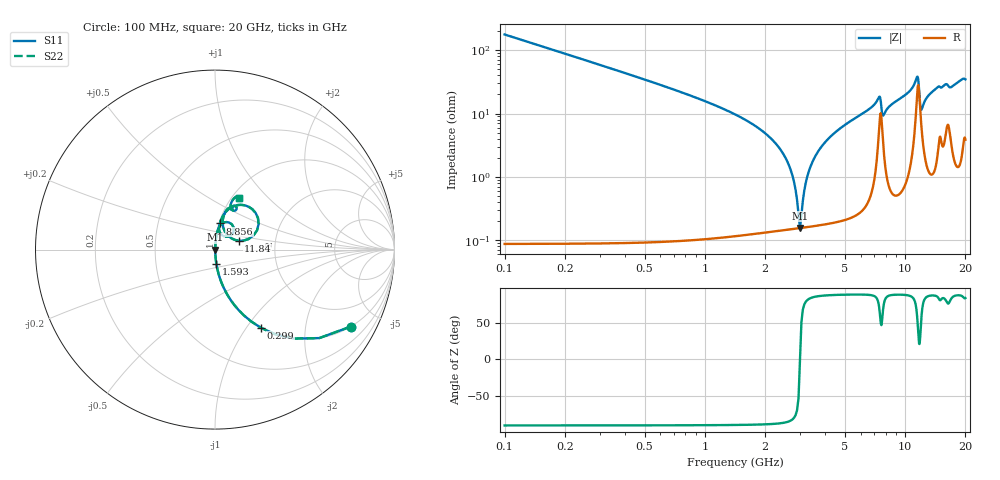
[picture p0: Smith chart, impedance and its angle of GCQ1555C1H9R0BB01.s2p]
!Murata Part Number: GCQ1555C1H9R0BB01
!These Parameters are Measured in Series Mode Connection
!Data Generated on Mar 13, 2026
!  o--ll--o
!Port1  Port2
!  o------o
!Operation Temp=25[degC], DC Bias Voltage=0[V]
!Freq. Start=100[MHz] Stop=20[GHz] 401[Steps]
# Hz S RI R 50
!Freq.(Hz) S11(Real) S11(Imag) S21(Real) S21(Imag) S12(Real) S12(Imag) S22(Real) S22(Imag)
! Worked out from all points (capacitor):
!   401 points, 100 MHz to 20 GHz, reference 50 ohm
!   read as one part in series: C = 9 pF near 199.5 MHz
!   lowest |Z| = 156 mohm at 2.986 GHz (marker M1)
!   series resonance near 2.987 GHz, so ESL is about 320 pH
!   S11 on the Smith chart (normalised r, x): 100 MHz: 1.00, -3.53; 299 MHz: 1.00, -1.17; 1.593 GHz: 1.00, -0.16; 8.856 GHz: 1.01, +0.30; 11.84 GHz: 1.30, +0.13; 20 GHz: 1.08, +0.69
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1e8  0.7572 -0.4285  0.2428 0.4285  0.2428 0.4285  0.7572 -0.4285
2.99e8  0.2556 -0.4354  0.7444 0.4354  0.7444 0.4354  0.2556 -0.4354
6.4725e8  0.0643 -0.2434  0.9357 0.2434  0.9357 0.2434  0.0643 -0.2434
1.5925e9  0.00747 -0.0788  0.9925 0.0788  0.9925 0.0788  0.00747 -0.0788
2.53775e9  0.00183 -0.0194  0.9982 0.0194  0.9982 0.0194  0.00183 -0.0194
2.73675e9  0.00161 -0.0104  0.9984 0.0104  0.9984 0.0104  0.00161 -0.0104
2.9855e9  0.00156 -4.39e-05  0.9984 4.39e-05  0.9984 4.39e-05  0.00156 -4.39e-05
3.085e9  0.00159 0.00385  0.9984 -0.00385  0.9984 -0.00385  0.00159 0.00385
3.23425e9  0.0017 0.00949  0.9983 -0.00949  0.9983 -0.00949  0.0017 0.00949
3.43325e9  0.00193 0.0167  0.9981 -0.0167  0.9981 -0.0167  0.00193 0.0167
4.478e9  0.00443 0.0501  0.9956 -0.0501  0.9956 -0.0501  0.00443 0.0501
6.7665e9  0.0203 0.121  0.9797 -0.121  0.9797 -0.121  0.0203 0.121
7.41325e9  0.0786 0.151  0.9214 -0.151  0.9214 -0.151  0.0786 0.151
7.7615e9  0.0404 0.0794  0.9596 -0.0794  0.9596 -0.0794  0.0404 0.0794
8.856e9  0.0269 0.1457  0.9731 -0.1457  0.9731 -0.1457  0.0269 0.1457
1.005e10  0.0445 0.1877  0.9555 -0.1877  0.9555 -0.1877  0.0445 0.1877
1.1443e10  0.2077 0.2254  0.7923 -0.2254  0.7923 -0.2254  0.2077 0.2254
1.1841e10  0.1316 0.0494  0.8684 -0.0494  0.8684 -0.0494  0.1316 0.0494
1.204e10  0.0699 0.0806  0.9301 -0.0806  0.9301 -0.0806  0.0699 0.0806
1.338325e10  0.0507 0.1943  0.9493 -0.1943  0.9493 -0.1943  0.0507 0.1943
1.67165e10  0.0996 0.218  0.9004 -0.218  0.9004 -0.218  0.0996 0.218
2e10  0.1322 0.287  0.8678 -0.287  0.8678 -0.287  0.1322 0.287
